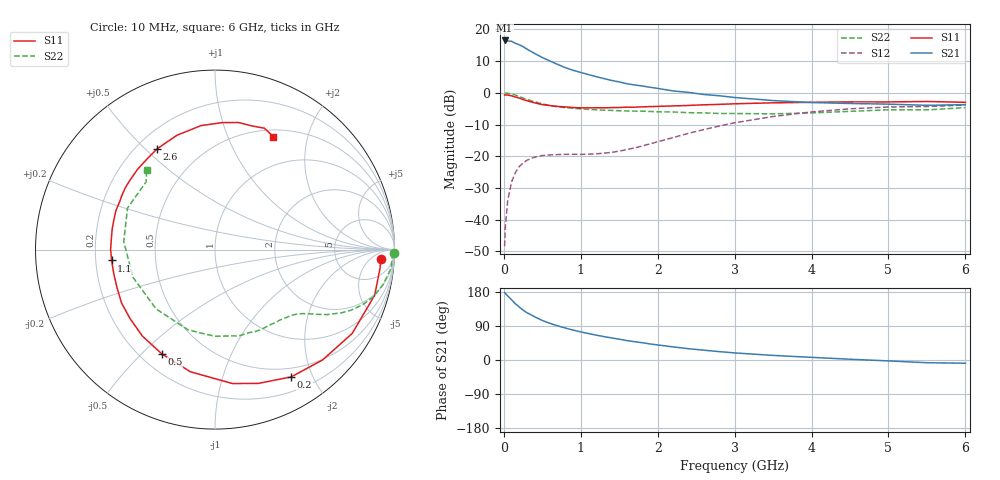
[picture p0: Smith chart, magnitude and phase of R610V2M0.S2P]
! SIEMENS Small Signal Semiconductors
! BFR193
! Si NPN RF Bipolar Junction Transistor in SOT23
! VCE = 10 V  IC = 2 mA
! Common Emitter S-Parameters:  May  1996
# GHz  S  MA  R  50
!  f  S11  S21  S12  S22
! GHz  MAG  ANG  MAG  ANG  MAG  ANG  MAG  ANG
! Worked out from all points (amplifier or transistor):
!   36 points, 10 MHz to 6 GHz, reference 50 ohm
!   highest |S21| = 16.5 dB at 10 MHz (marker M1)
!   |S21| within 3 dB of that: start of sweep to 319.5 MHz
!   unconditionally stable (mu >= 1): 1.173 GHz to 2.046 GHz
!   at 250 MHz: K = 0.23, MSG = 18.4 dB, |S12| = -22.2 dB
!   at 1.4 GHz: K = 1.11, MAG = 9.4 dB, |S12| = -18.8 dB
!   at 6 GHz: K = 0.99, MSG = 0.1 dB, |S12| = -3.9 dB
!   S11 on the Smith chart (normalised r, x): 10 MHz: 17, -12; 200 MHz: 0.38, -1.70; 500 MHz: 0.28, -0.57; 1.1 GHz: 0.27, -0.05; 2.6 GHz: 0.28, +0.54; 6 GHz: 0.58, +1.48
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0.01  0.9255 -3.2  6.708 178.1  0.0038 84.1  0.9963 -1.2
0.02  0.9254 -6.3  6.595 175.5  0.0078 86.1  0.9883 -2.4
0.05  0.9254 -15.9  6.591 169.2  0.0198 81.0  0.9868 -6.0
0.1  0.8959 -31.4  6.504 159.0  0.0391 72.9  0.9574 -11.6
0.15  0.8587 -45.7  6.047 148.5  0.0551 65.0  0.9214 -16.6
0.2  0.8265 -59.1  5.744 139.9  0.0684 58.7  0.8775 -20.5
0.25  0.7835 -72.1  5.359 131.6  0.078 53.1  0.8285 -24.1
0.3  0.7525 -82.6  4.897 125.0  0.0863 48.6  0.7869 -26.6
0.4  0.6943 -101.4  4.185 114.1  0.0968 41.6  0.722 -30.1
0.5  0.6521 -117.1  3.61 104.3  0.1025 37.3  0.6689 -32.6
0.6  0.629 -130.1  3.176 96.7  0.1046 35.0  0.6292 -34.6
0.7  0.6096 -140.9  2.807 90.1  0.106 33.6  0.6026 -36.3
0.9  0.5857 -158.7  2.267 79.0  0.1074 34.0  0.5706 -39.5
1.1  0.579 -174.0  1.939 69.8  0.1077 38.2  0.5483 -43.6
1.3  0.5805 174.0  1.679 61.8  0.1119 44.4  0.5323 -47.9
1.6  0.5932 158.7  1.391 51.2  0.127 54.1  0.5175 -55.5
2.2  0.6215 134.1  1.072 34.6  0.1965 64.4  0.499 -74.4
2.6  0.6471 120.0  0.941 25.9  0.2631 63.2  0.4826 -90.1
3.5  0.6953 96.4  0.755 12.1  0.4231 48.7  0.4658 -134.8
4.5  0.72 79.6  0.679 2.0  0.56 27.8  0.5102 175.1
5.5  0.73 67.9  0.635 -7.2  0.6075 8.1  0.5383 135.5
6  0.7089 62.7  0.651 -8.5  0.6414 2.8  0.5839 130.7
